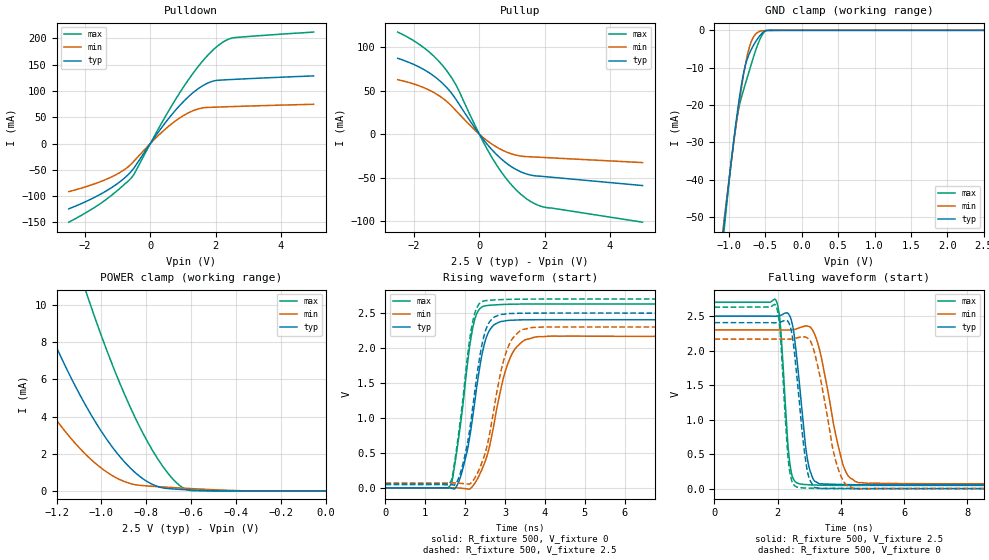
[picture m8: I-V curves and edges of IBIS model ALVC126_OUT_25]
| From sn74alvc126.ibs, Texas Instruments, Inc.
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[Model]   ALVC126_OUT_25
Model_type  3-state
Enable   Active-High
Vref =   0
Rref =   500
Cref =   30p
Vmeas =   1.25
| variable   typ   min   max
C_comp   5.13pF   4.44pF   5.92pF
| C_pullup   6.21pF   5.05pF   6.85pF
| C_pulldown   8.67pF   5.01pF   13.48pF
| C_tri-state   5.13pF   4.44pF   5.92pF
[Temperature Range]   40   100   -40
| Ambient temperature   25   85   -40
[Voltage range]   2.5   2.3   2.7
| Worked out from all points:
|   slope of the pulldown table from 0 to 0.375 V, typ, clamps not added: 11.5 ohm
|   slope of the pullup table from 0 to 0.375 V, typ, clamps not added: 21.5 ohm
|   GND clamp passes 1 mA (typ) near -0.56 V on its own axis
|   POWER clamp passes 1 mA (typ) near -0.85 V on its own axis
|   rising waveform, R_fixture 500, V_fixture 0: 20-80 % time 396ps typ, 509ps min, 344ps max; typ from 0 V to 2.4 V
|   falling waveform, R_fixture 500, V_fixture 2.5: 20-80 % time 326ps typ, 568ps min, 219ps max; typ from 2.5 V to 0.054 V
|   rising waveform, R_fixture 500, V_fixture 2.5: 20-80 % time 384ps typ, 471ps min, 338ps max; typ from 0.054 V to 2.5 V
|   falling waveform, R_fixture 500, V_fixture 0: 20-80 % time 321ps typ, 531ps min, 210ps max; typ from 2.4 V to 0 V
[GND Clamp]
| ALVC126_OUT_25
|   Voltage   I(typ)   I(min)   I(max)
-2.5V     -335.9mA   -310.3mA   -363.5mA
-1.085V   -55.14mA   -53.69mA   -56.9mA
-1.065V   -51.58mA   -50.43mA   -53.01mA
-1.05V    -48.93mA   -48.01mA   -50.13mA
-960mV    -33.57mA   -33.87mA   -33.74mA
-900mV    -24.12mA   -24.99mA   -24.7mA
-810mV    -12.48mA   -13.09mA   -16.62mA
-765mV    -8.677mA   -8.228mA   -13.67mA
-705mV    -5.559mA   -3.602mA   -9.787mA
-590mV    -1.784mA   -364.8uA   -3.068mA
-480mV    -21.04uA   -62.18uA   -16.51uA
2.5V      76.41pA    70.77nA    33.05pA
[POWER Clamp]
| ALVC126_OUT_25
|   Voltage   I(typ)   I(min)   I(max)
-2.5V     60.05mA    40.54mA    89.37mA
-1.535V   18.19mA    10.69mA    31.45mA
-1.515V   17.49mA    10.21mA    30.43mA
-1.295V   10.36mA    5.473mA    19.9mA
-1.165V   6.812mA    3.253mA    14.39mA
-1.06V    4.383mA    1.846mA    10.4mA
-950mV    2.335mA    812.2uA    6.743mA
-845mV    938.6uA    325.5uA    3.823mA
-745mV    219.5uA    228.1uA    1.65mA
-655mV    86.61uA    162.8uA    329uA
-595mV    47.87uA    122.3uA    14.43uA
-31.15fV  76.41pA    373.2pA    35.97pA
[Pulldown]
| ALVC126_OUT_25
|   Voltage   I(typ)   I(min)   I(max)
-2.5V     -124.2mA   -91.47mA   -149.5mA
-1.32V    -88.93mA   -67.13mA   -104.8mA
-885mV    -70.36mA   -53.26mA   -82.59mA
-580mV    -52.49mA   -38.64mA   -65.21mA
310mV     27.29mA    19.1mA     35.11mA
975mV     77.23mA    51.61mA    103.6mA
1.575V    108.7mA    67.33mA    154.7mA
1.845V    117mA      68.73mA    173.2mA
2.09V     120.3mA    69.29mA    186.8mA
2.335V    121.1mA    69.82mA    196.5mA
2.56V     121.8mA    70.29mA    201.1mA
5V        128.5mA    74.54mA    211.7mA
[Pullup]
| ALVC126_OUT_25
|   Voltage   I(typ)   I(min)   I(max)
-2.5V     87.37mA    62.76mA    117.6mA
-1.665V   73.65mA    52.98mA    98.57mA
-1.325V   64.98mA    46.46mA    87.24mA
-1.025V   54.72mA    38.5mA     74.32mA
-680mV    38mA       25.67mA    54.12mA
30mV      -1.546mA   -1.013mA   -2.276mA
440mV     -20.07mA   -12.77mA   -30.18mA
910mV     -35.58mA   -21.66mA   -55.12mA
1.38V     -44.98mA   -25.67mA   -72.55mA
1.69V     -47.85mA   -26.28mA   -79.94mA
2.005V    -48.85mA   -26.89mA   -84.12mA
5V        -59.15mA   -32.69mA   -101.3mA
[Ramp]
| ALVC126_OUT_25
| variable   typ   min   max
dV/dt_r   1.45/4.08E-10   1.31/5.28E-10   1.58/3.49E-10
dV/dt_f   1.50/3.45E-10   1.37/6.09E-10   1.62/2.32E-10
R_load = 500
[Rising Waveform]
| ALVC126_OUT_25
R_fixture =   500
C_fixture =   0
L_fixture =   0
V_fixture =   0
V_fixture_min = 0
V_fixture_max = 0
|   Time   V(typ)   V(min)   V(max)
0s        28.66pV    2.142nV    22.86pV
1.65ns    -5.755mV   1.455mV    54.88mV
1.905ns   197.6mV    -5.079mV   1.006V
2.2ns     1.055V     31.15mV    2.313V
2.415ns   1.885V     255.8mV    2.583V
2.61ns    2.253V     590.7mV    2.611V
2.945ns   2.384V     1.539V     2.623V
3.14ns    2.398V     1.873V     2.627V
3.85ns    2.405V     2.163V     2.63V
50ns      2.405V     2.167V     2.63V
[Falling Waveform]
| ALVC126_OUT_25
R_fixture =   500
C_fixture =   0
L_fixture =   0
V_fixture =   2.5
V_fixture_min = 2.3
V_fixture_max = 2.7
|   Time   V(typ)   V(min)   V(max)
0s        2.5V       2.3V       2.7V
1.955ns   2.499V     2.3V       2.721V
2.085ns   2.51V      2.299V     2.367V
2.395ns   2.49V      2.299V     335.7mV
2.53ns    2.199V     2.305V     113.1mV
2.815ns   925.3mV    2.35V      60.12mV
3.165ns   110.7mV    2.243V     51.57mV
4.065ns   59.28mV    347.3mV    45.68mV
4.58ns    55.17mV    84.65mV    45.32mV
50ns      53.74mV    69.35mV    45.86mV
[Rising Waveform]
| ALVC126_OUT_25
R_fixture =   500
C_fixture =   0
L_fixture =   0
V_fixture =   2.5
V_fixture_min = 2.3
V_fixture_max = 2.7
|   Time   V(typ)   V(min)   V(max)
0s        53.74mV    69.35mV    45.86mV
1.65ns    47.94mV    70.54mV    101.7mV
1.9ns     249.4mV    64.05mV    1.064V
2.18ns    1.112V     91.23mV    2.348V
2.39ns    1.956V     316.3mV    2.651V
2.54ns    2.294V     576.9mV    2.68V
2.89ns    2.479V     1.647V     2.692V
3.07ns    2.492V     2.002V     2.696V
3.705ns   2.5V       2.295V     2.7V
50ns      2.5V       2.3V       2.7V
[Falling Waveform]
| ALVC126_OUT_25
R_fixture =   500
C_fixture =   0
L_fixture =   0
V_fixture =   0
V_fixture_min = 0
V_fixture_max = 0
|   Time   V(typ)   V(min)   V(max)
0s        2.405V     2.167V     2.63V
1.95ns    2.404V     2.167V     2.643V
2.075ns   2.413V     2.166V     2.291V
2.365ns   2.39V      2.167V     300.7mV
2.705ns   1.161V     2.194V     13.34mV
2.915ns   313.7mV    2.189V     7.589mV
3.125ns   42.11mV    2.035V     4.18mV
3.89ns    3.464mV    319.6mV    -156.2uV
4.505ns   831.3uV    -8.513mV   -462.1uV
50ns      -9.529nV   7.53nV     -12.11nV
